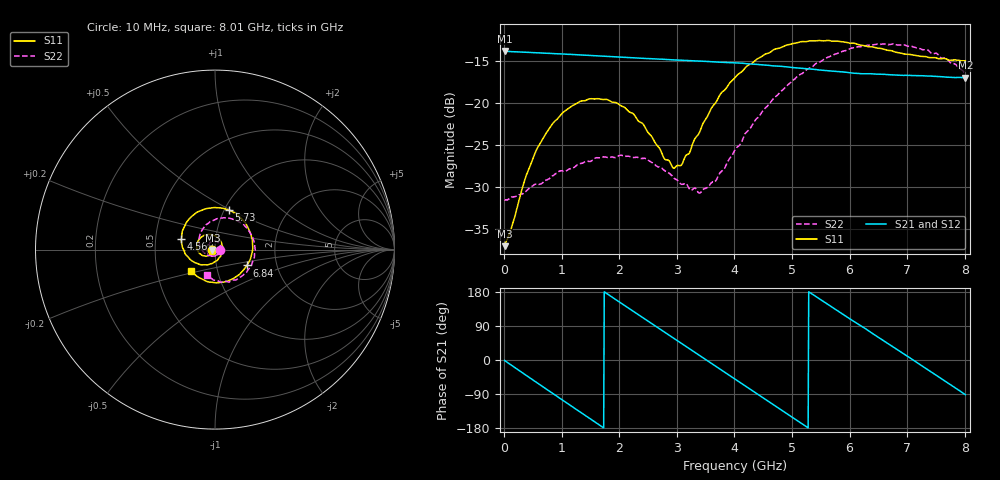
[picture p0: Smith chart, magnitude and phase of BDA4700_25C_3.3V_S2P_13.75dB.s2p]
!Agilent Technologies,E5071B,MY42404982,A.09.10
!Date: Mon Oct 20 18:08:48 2025
!Data & Calibration Information:
!Freq	S11:SOLT2(ON)	S21:SOLT2(ON)	S12:SOLT2(ON)	S22:SOLT2(ON)
# Hz S RI R 50
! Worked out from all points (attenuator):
!   801 points, 10 MHz to 8.01 GHz, reference 50 ohm
!   highest |S21| = -13.85 dB at 10 MHz (marker M1); lowest = -17.0 dB at 8.01 GHz (marker M2)
!   lowest |S11| = -37.0 dB at 10 MHz (marker M3), VSWR 1.03, Z = 48.6 - j0.137 ohm
!   |S11| at or under -10 dB: start of sweep to end of sweep
!   |S22| runs from -31.6 to -13.0 dB; largest |S21 - S12| = 0.0024
!   S11 on the Smith chart (normalised r, x): 10 MHz: 0.97, -0.00; 4.56 GHz: 0.68, +0.08; 5.73 GHz: 1.05, +0.49; 6.84 GHz: 1.41, -0.26; 8.01 GHz: 0.75, -0.18
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1e7  -0.014 -0.0014  0.2029 -0.0044  0.2028 -0.00464  0.0266 -0.000982
3.7e8  -0.0245 -0.0259  0.1553 -0.1256  0.1552 -0.1256  0.0219 -0.0198
5.9e8  -0.0415 -0.0357  0.0936 -0.1747  0.0935 -0.1746  0.0132 -0.0302
1e9  -0.0822 -0.0244  -0.0476 -0.1891  -0.0475 -0.1893  -0.0176 -0.0353
1.35e9  -0.1019 0.0123  -0.1477 -0.1232  -0.1478 -0.1234  -0.0409 -0.0154
1.71e9  -0.0868 0.0585  -0.1892 -0.00984  -0.1894 -0.00976  -0.045 0.0156
2.07e9  -0.0432 0.0843  -0.1551 0.1037  -0.1552 0.1038  -0.0254 0.0411
2.68e9  0.0348 0.0424  0.0177 0.1811  0.0174 0.181  0.0239 0.034
2.93e9  0.0412 0.00225  0.0922 0.1547  0.0921 0.1543  0.0327 0.0158
3.07e9  0.0366 -0.0214  0.1271 0.1263  0.1258 0.1272  0.0329 0.0031
3.42e9  -0.00517 -0.0703  0.1743 0.0298  0.1745 0.0299  0.017 -0.024
3.67e9  -0.0523 -0.0847  0.1686 -0.0471  0.1686 -0.0474  -0.00469 -0.034
4.01e9  -0.1258 -0.064  0.1108 -0.1327  0.111 -0.1323  -0.0435 -0.0293
4.56e9  -0.1873 0.0575  -0.0464 -0.1607  -0.0461 -0.1609  -0.0875 0.0362
4.98e9  -0.1438 0.1707  -0.1386 -0.0845  -0.1388 -0.0853  -0.0701 0.1123
5.35e9  -0.0455 0.2285  -0.1575 0.0167  -0.1576 0.0158  -0.00754 0.1632
5.73e9  0.0772 0.2193  -0.1108 0.107  -0.1107 0.107  0.086 0.1735
6.23e9  0.1918 0.1062  0.00826 0.1485  0.0103 0.1484  0.1939 0.0961
6.68e9  0.2007 -0.0401  0.1093 0.0982  0.1097 0.098  0.221 -0.0238
6.84e9  0.1782 -0.088  0.131 0.0644  0.1315 0.0634  0.2096 -0.0673
7.45e9  0.0162 -0.185  0.1178 -0.0824  0.1179 -0.0827  0.0881 -0.1745
8.01e9  -0.1325 -0.1186  -0.00395 -0.1409  -0.00344 -0.141  -0.046 -0.1434
